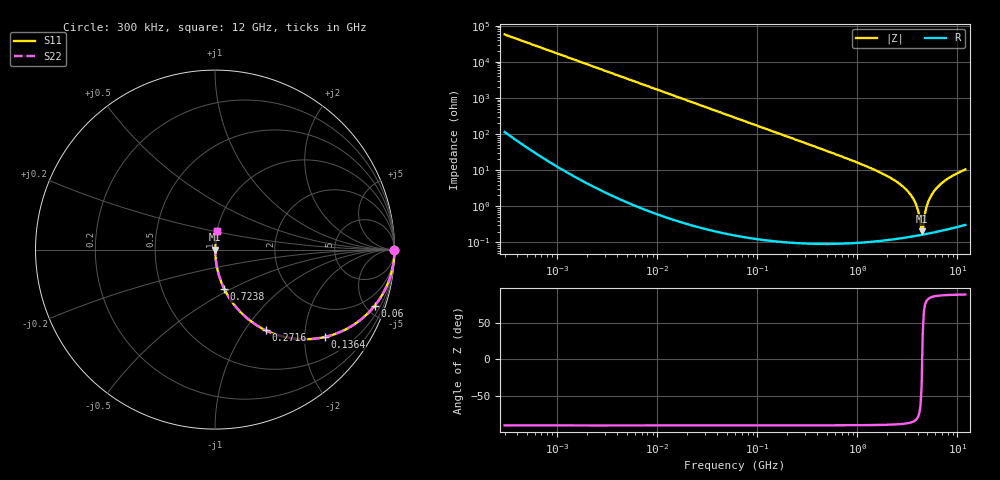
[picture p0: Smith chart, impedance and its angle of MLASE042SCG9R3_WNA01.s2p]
! MLASE042SCG9R3_WNA01  S-PARAMETER MODEL  ( General Type )
! Model Generated by TAIYO YUDEN Corporation (http://www.ty-top.com)
! Version 1.0
! TAIYO YUDEN Control No. 130801
! Copyright(c) 2013 TAIYO YUDEN CO.,LTD. All Rights Reserved.
! Product Description (link to TY-COMPAS)
! https://ds.yuden.co.jp/TYCOMPAS/or/detail?pn=MLASE042SCG9R3BWNA01&u=M
! Products Name : Multilayer Ceramic Capacitors
! Characteristics :
!  Capacitance : 9.3 pF , Rated Voltage : 16V , TCC : CG / C0G
!  Case Size : 0.4 x 0.2 / 0.016 x 0.008 [mm/inch] , Thickness : 0.2 / 0.008 [mm/inch]
!  (Conditions: Temperature = 25 degC , DC Bias Current/Voltage = 0A / 0V)
! External Node Assignments :
!  1  o---| |---o  2
! GND o---------o GND
! Frequency Range : 0.3MHz  -  12000MHz  [ 401 STEP ]
# MHz S RI R 50
! Freq[MHz].  S11 Real  S11 Imag  S21 Real  S21 Imag  S12 Real  S12 Imag  S22 Real  S22 Imag
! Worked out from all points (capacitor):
!   401 points, 300 kHz to 12 GHz, reference 50 ohm
!   read as one part in series: C = 9.28 pF near 316.3 kHz
!   lowest |Z| = 203 mohm at 4.385 GHz (marker M1)
!   series resonance near 4.443 GHz, so ESL is about 140 pH
!   S11 on the Smith chart (normalised r, x): 300 kHz: open; 60 MHz: 1.00, -5.71; 136.4 MHz: 1.00, -2.51; 271.6 MHz: 1.00, -1.26; 723.8 MHz: 1.00, -0.46; 12 GHz: 1.01, +0.21
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0.3  1 -0.00175  6.56e-06 0.00175  6.56e-06 0.00175  1 -0.00175
1.769972  0.9999 -0.0103  0.000112 0.0103  0.000112 0.0103  0.9999 -0.0103
10.44266  0.9963 -0.0607  0.00372 0.0607  0.00372 0.0607  0.9963 -0.0607
26.39317  0.9768 -0.1504  0.0232 0.1504  0.0232 0.1504  0.9768 -0.1504
60  0.8907 -0.3117  0.1093 0.3117  0.1093 0.3117  0.8907 -0.3117
136.3989  0.6118 -0.4869  0.3882 0.4869  0.3882 0.4869  0.6118 -0.4869
271.6094  0.2837 -0.45  0.7163 0.45  0.7163 0.45  0.2837 -0.45
353.9943  0.1885 -0.3901  0.8115 0.3901  0.8115 0.3901  0.1885 -0.3901
723.8279  0.0513 -0.2186  0.9487 0.2186  0.9487 0.2186  0.0513 -0.2186
2088.533  0.00525 -0.0636  0.9948 0.0636  0.9948 0.0636  0.00525 -0.0636
2795.104  0.00269 -0.037  0.9973 0.037  0.9973 0.037  0.00269 -0.037
3454.93  0.00183 -0.0197  0.9982 0.0197  0.9982 0.0197  0.00183 -0.0197
3841.137  0.00165 -0.0114  0.9983 0.0114  0.9983 0.0114  0.00165 -0.0114
4050.141  0.00161 -0.00728  0.9984 0.00728  0.9984 0.00728  0.00161 -0.00728
4270.516  0.00161 -0.0032  0.9984 0.0032  0.9984 0.0032  0.00161 -0.0032
4385.161  0.00163 -0.00121  0.9984 0.00121  0.9984 0.00121  0.00163 -0.00121
4623.766  0.00168 0.00366  0.9983 -0.00366  0.9983 -0.00366  0.00168 0.00366
4875.354  0.00179 0.00866  0.9982 -0.00866  0.9982 -0.00866  0.00179 0.00866
5140.631  0.00196 0.0137  0.998 -0.0137  0.998 -0.0137  0.00196 0.0137
6026.253  0.0028 0.0293  0.9972 -0.0293  0.9972 -0.0293  0.0028 0.0293
8064.993  0.0058 0.0588  0.9942 -0.0588  0.9942 -0.0588  0.0058 0.0588
12000  0.0139 0.1032  0.9861 -0.1032  0.9861 -0.1032  0.0139 0.1032
